| IBIS file stm32f373_378_383_lqfp48.ibs
[IBIS ver] 4.2
[File name] stm32f373_378_383_lqfp48.ibs
[File Rev] 1.0
[Date]  29-09-2025
[Source] Data Created at STMicroelectronics
[Notes]  File originated from ELDO simulations.
[Disclaimer]  This information is for modeling purpose only and is
   not guaranted. The information is subject to change without
   notice.
[Copyright] Copyright 2025 STMicroelectronics Inc.
|   Component stm32f373_378_383_lqfp48
[Component] stm32f373_378_383_lqfp48
[Manufacturer] STMicroelectronics
[Package]
| variable   typ   min   max
R_pkg  0  NA  NA
L_pkg  0  NA  NA
C_pkg  0  NA  NA
[Pin]   signal_name   model_name R_pin  L_pin C_pin
1 VBAT POWER 0.053 3.42534E-09 9.041E-14
2 PC13-WKUP2 io8p_sudq_tc_v33 0.048377332 2.91404E-09 6.443E-14
3 PC14-OSC32IN io8p_sudq_tc_v33 0.044678997 2.50442E-09 4.365E-14
4 PC15-OSC32OUT io8p_sudq_tc_v33 0.041905328 2.19704E-09 2.807E-14
5 PF0/OSC_IN io8p_wsudqh_i2c_ft 0.040056325 1.9919E-09 1.769E-14
6 PF1/OSC_OUT io8p_wsudqh_i2c_ft 0.03913 1.89021E-09 1.24625E-14
7 NRST ioreset_tc_v33 0.03913 1.89021E-09 1.24625E-14
8 VSSA/VREF- GND 0.040057312 1.98992E-09 1.775E-14
9 VDDA/VREF+ POWER 0.041906973 2.19374E-09 2.817E-14
10 PA0 io8p_sudq_ft 0.0446813 2.4998E-09 4.379E-14
11 PA1 io8p_sudq_ft 0.048380293 2.9081E-09 6.461E-14
12 PA2 io8p_sudq_ft 0.053 3.42534E-09 9.041E-14
13 PA3 io8p_sudq_ft 0.053 3.42534E-09 9.041E-14
14 PA4 io8p_sudq_ft 0.048377332 2.91404E-09 6.443E-14
15 PA5 io8p_sudq_ft 0.044678997 2.50442E-09 4.365E-14
16 PA6 io8p_sudq_ft 0.041905328 2.19704E-09 2.807E-14
17 VDD POWER 0.040056325 1.9919E-09 1.769E-14
18 PB0 io8p_sudq_ft 0.03913 1.89021E-09 1.24625E-14
19 PB1 io8p_sudq_ft 0.03913 1.89021E-09 1.24625E-14
20 PB2 io8p_sudq_ft 0.040057312 1.98992E-09 1.775E-14
21 PE8 io8p_sudq_ft 0.041906973 2.19374E-09 2.817E-14
22 PE9 io8p_sudq_ft 0.0446813 2.4998E-09 4.379E-14
23 VSSSD/VREFSD- GND 0.048380293 2.9081E-09 6.461E-14
24 VDDSD POWER 0.053 3.42534E-09 9.041E-14
25 REFSD+ POWER 0.053 3.42534E-09 9.041E-14
26 PB14 io8p_sudq_ft 0.048377332 2.91404E-09 6.443E-14
27 PB15 io8p_sudq_ft 0.044678997 2.50442E-09 4.365E-14
28 PD8 io8p_sudq_ft 0.041905328 2.19704E-09 2.807E-14
29 PA8 io8p_sudq_ft 0.040056325 1.9919E-09 1.769E-14
30 PA9 io8p_wsudqh_i2c_ft 0.03913 1.89021E-09 1.24625E-14
31 PA10 io8p_wsudqh_i2c_ft 0.03913 1.89021E-09 1.24625E-14
32 PA11 io8usb_lv_ft 0.040057312 1.98992E-09 1.775E-14
33 PA12 io8usb_lv_ft 0.041906973 2.19374E-09 2.817E-14
34 PA13 io8p_sudq_ft 0.0446813 2.4998E-09 4.379E-14
35 PF6 io8p_wsudqh_i2c_ft 0.048380293 2.9081E-09 6.461E-14
36 PF7 io8p_wsudqh_i2c_ft 0.053 3.42534E-09 9.041E-14
37 PA14 io8p_wsudqh_i2c_ft 0.053 3.42534E-09 9.041E-14
38 PA15 io8p_wsudqh_i2c_ft 0.048377332 2.91404E-09 6.443E-14
39 PB3 io8p_sudq_ft 0.044678997 2.50442E-09 4.365E-14
40 PB4 io8p_sudq_ft 0.041905328 2.19704E-09 2.807E-14
41 PB5 io8p_sudq_ft 0.040056325 1.9919E-09 1.769E-14
42 PB6 io8p_wsudqh_i2c_ft 0.03913 1.89021E-09 1.24625E-14
43 PB7 io8p_wsudqh_i2c_ft 0.03913 1.89021E-09 1.24625E-14
44 BOOT0 vpp_test_hv 0.040057312 1.98992E-09 1.775E-14
45 PB8 io8p_wsudqh_i2c_ft 0.041906973 2.19374E-09 2.817E-14
46 PB9 io8p_wsudqh_i2c_ft 0.0446813 2.4998E-09 4.379E-14
47 VSS GND 0.048380293 2.9081E-09 6.461E-14
48 VDD POWER 0.053 3.42534E-09 9.041E-14
[Model Selector] io8p_sudq_ft
io8p01_sudq_ft_pd_lv  "SPEED01 2P0V, PD=40kOhm"
io8p01_sudq_ft_pu_lv  "SPEED01 2P0V, PU=40kOhm"
io8p01_sudq_ft_lv  "SPEED01 2P0V"
io8p10_sudq_ft_pd_lv  "SPEED10 2P0V, PD=40kOhm"
io8p10_sudq_ft_pu_lv  "SPEED10 2P0V, PU=40kOhm"
io8p10_sudq_ft_lv  "SPEED10 2P0V"
io8p11_sudq_ft_pd_lv  "SPEED11 2P0V, PD=40kOhm"
io8p11_sudq_ft_pu_lv  "SPEED11 2P0V, PU=40kOhm"
io8p11_sudq_ft_lv  "SPEED11 2P0V"
io8p01_sudq_ft_pd  "SPEED01, PD=40kOhm"
io8p01_sudq_ft_pu  "SPEED01, PU=40kOhm"
io8p01_sudq_ft  "SPEED01"
io8p10_sudq_ft_pd  "SPEED10, PD=40kOhm"
io8p10_sudq_ft_pu  "SPEED10, PU=40kOhm"
io8p10_sudq_ft  "SPEED10"
io8p11_sudq_ft_pd  "SPEED11, PD=40kOhm"
io8p11_sudq_ft_pu  "SPEED11, PU=40kOhm"
io8p11_sudq_ft  "SPEED11"
[Model Selector] io8p_sudq_tc_v33
io8p01_sudq_tc_v33_pd_lv  "SPEED01 2P0V, PD=40kOhm"
io8p01_sudq_tc_v33_pu_lv  "SPEED01 2P0V, PU=40kOhm"
io8p01_sudq_tc_v33_lv  "SPEED01 2P0V"
io8p10_sudq_tc_v33_pd_lv  "SPEED10 2P0V, PD=40kOhm"
io8p10_sudq_tc_v33_pu_lv  "SPEED10 2P0V, PU=40kOhm"
io8p10_sudq_tc_v33_lv  "SPEED10 2P0V"
io8p11_sudq_tc_v33_pd_lv  "SPEED11 2P0V, PD=40kOhm"
io8p11_sudq_tc_v33_pu_lv  "SPEED11 2P0V, PU=40kOhm"
io8p11_sudq_tc_v33_lv  "SPEED11 2P0V"
io8p01_sudq_tc_v33_pd  "SPEED01, PD=40kOhm"
io8p01_sudq_tc_v33_pu  "SPEED01, PU=40kOhm"
io8p01_sudq_tc_v33  "SPEED01"
io8p10_sudq_tc_v33_pd  "SPEED10, PD=40kOhm"
io8p10_sudq_tc_v33_pu  "SPEED10, PU=40kOhm"
io8p10_sudq_tc_v33  "SPEED10"
io8p11_sudq_tc_v33_pd  "SPEED11, PD=40kOhm"
io8p11_sudq_tc_v33_pu  "SPEED11, PU=40kOhm"
io8p11_sudq_tc_v33  "SPEED11"
[Model Selector] io8p_wsudqh_i2c_ft
io8p_wsudqh_i2c_ft_lv_pd  "General purpose IO with I2C capability on. 5V tolerant. 1.8V range with pull down"
io8p_wsudqh_i2c_ft_lv_pu  "General purpose IO with I2C capability on. 5V tolerant. 1.8V range with pull up"
io8p_wsudqh_i2c_ft_lv  "General purpose IO with I2C capability on. 5V tolerant. 1.8V range"
io8p_wsudqh_i2c_ft_pd  "General purpose IO with I2C capability on. 5V tolerant. 3.3V range with pull down"
io8p_wsudqh_i2c_ft_pu  "General purpose IO with I2C capability on. 5V tolerant. 3.3V range with pull up"
io8p_wsudqh_i2c_ft_i2c  "General purpose IO with I2C capability on. 5V tolerant. 3.3V range"
[Model Selector] io8usb_lv_ft
io8usb_dpdn_lv_ft_pd  "FS USB DP/DN IO + PD=40kOhm"
io8usb_dpdn_lv_ft_pu  "FS USB DP/DN IO + PU=40kOhm"
io8usb_dpdn_lv_ft  "FS USB DP/DN IO"
io8p01_lv_ft_pd_lv  "SPEED01 2P0V, PD=40kOhm"
io8p01_lv_ft_pu_lv  "SPEED01 2P0V, PU=40kOhm"
io8p01_lv_ft_lv  "SPEED01 2P0V"
io8p10_lv_ft_pd_lv  "SPEED10 2P0V, PD=40kOhm"
io8p10_lv_ft_pu_lv  "SPEED10 2P0V, PU=40kOhm"
io8p10_lv_ft_lv  "SPEED10 2P0V"
io8p11_lv_ft_pd_lv  "SPEED11 2P0V, PD=40kOhm"
io8p11_lv_ft_pu_lv  "SPEED11 2P0V, PU=40kOhm"
io8p11_lv_ft_lv  "SPEED11 2P0V"
io8p01_lv_ft_pd  "SPEED01, PD=40kOhm"
io8p01_lv_ft_pu  "SPEED01, PU=40kOhm"
io8p01_lv_ft  "SPEED01"
io8p10_lv_ft_pd  "SPEED10, PD=40kOhm"
io8p10_lv_ft_pu  "SPEED10, PU=40kOhm"
io8p10_lv_ft  "SPEED10"
io8p11_lv_ft_pd  "SPEED11, PD=40kOhm"
io8p11_lv_ft_pu  "SPEED11, PU=40kOhm"
io8p11_lv_ft  "SPEED11"
[Model Selector] ioreset_tc_v33
ioreset_tc_v33_pu_lv  "IORESET 2V + PU=40kOhm"
ioreset_tc_v33_nopu_lv  "IORESET 2V"
ioreset_tc_v33_pu  "IORESET + PU=40kOhm"
ioreset_tc_v33_nopu  "IORESET"
[Model Selector] vpp_test_hv
vpp_test_hv_3p3  "Input Buffer"
vpp_test_hv_2p4  "Input Buffer 2P0V"
| Models and submodels in the file (69): io8p01_sudq_ft_pd_lv (I/O), io8p01_sudq_ft_pu_lv (I/O), io8p01_sudq_ft_lv (I/O), io8p10_sudq_ft_pd_lv (I/O), io8p10_sudq_ft_pu_lv (I/O), io8p10_sudq_ft_lv (I/O), io8p11_sudq_ft_pd_lv (I/O), io8p11_sudq_ft_pu_lv (I/O), io8p11_sudq_ft_lv (I/O), io8p01_sudq_ft_pd (I/O), io8p01_sudq_ft_pu (I/O), io8p01_sudq_ft (I/O), io8p10_sudq_ft_pd (I/O), io8p10_sudq_ft_pu (I/O), io8p10_sudq_ft (I/O), io8p11_sudq_ft_pd (I/O), io8p11_sudq_ft_pu (I/O), io8p11_sudq_ft (I/O), io8p01_sudq_tc_v33_pd_lv (I/O), io8p01_sudq_tc_v33_pu_lv (I/O), io8p01_sudq_tc_v33_lv (I/O), io8p10_sudq_tc_v33_pd_lv (I/O), io8p10_sudq_tc_v33_pu_lv (I/O), io8p10_sudq_tc_v33_lv (I/O), io8p11_sudq_tc_v33_pd_lv (I/O), io8p11_sudq_tc_v33_pu_lv (I/O), io8p11_sudq_tc_v33_lv (I/O), io8p01_sudq_tc_v33_pd (I/O), io8p01_sudq_tc_v33_pu (I/O), io8p01_sudq_tc_v33 (I/O), io8p10_sudq_tc_v33_pd (I/O), io8p10_sudq_tc_v33_pu (I/O), io8p10_sudq_tc_v33 (I/O), io8p11_sudq_tc_v33_pd (I/O), io8p11_sudq_tc_v33_pu (I/O), io8p11_sudq_tc_v33 (I/O), io8p_wsudqh_i2c_ft_lv_pd (I/O), io8p_wsudqh_i2c_ft_lv_pu (I/O), io8p_wsudqh_i2c_ft_lv (I/O), io8p_wsudqh_i2c_ft_pd (I/O), io8p_wsudqh_i2c_ft_pu (I/O), io8p_wsudqh_i2c_ft_i2c (I/O), io8usb_dpdn_lv_ft_pd (I/O), io8usb_dpdn_lv_ft_pu (I/O), io8usb_dpdn_lv_ft (I/O), io8p01_lv_ft_pd_lv (I/O), io8p01_lv_ft_pu_lv (I/O), io8p01_lv_ft_lv (I/O), io8p10_lv_ft_pd_lv (I/O), io8p10_lv_ft_pu_lv (I/O), io8p10_lv_ft_lv (I/O), io8p11_lv_ft_pd_lv (I/O), io8p11_lv_ft_pu_lv (I/O), io8p11_lv_ft_lv (I/O), io8p01_lv_ft_pd (I/O), io8p01_lv_ft_pu (I/O), io8p01_lv_ft (I/O), io8p10_lv_ft_pd (I/O), io8p10_lv_ft_pu (I/O), io8p10_lv_ft (I/O), io8p11_lv_ft_pd (I/O), io8p11_lv_ft_pu (I/O), io8p11_lv_ft (I/O), ioreset_tc_v33_pu_lv (I/O_open_drain), ioreset_tc_v33_nopu_lv (I/O_open_drain), ioreset_tc_v33_pu (I/O_open_drain), ioreset_tc_v33_nopu (I/O_open_drain), vpp_test_hv_2p4 (Input), vpp_test_hv_3p3 (Input)
